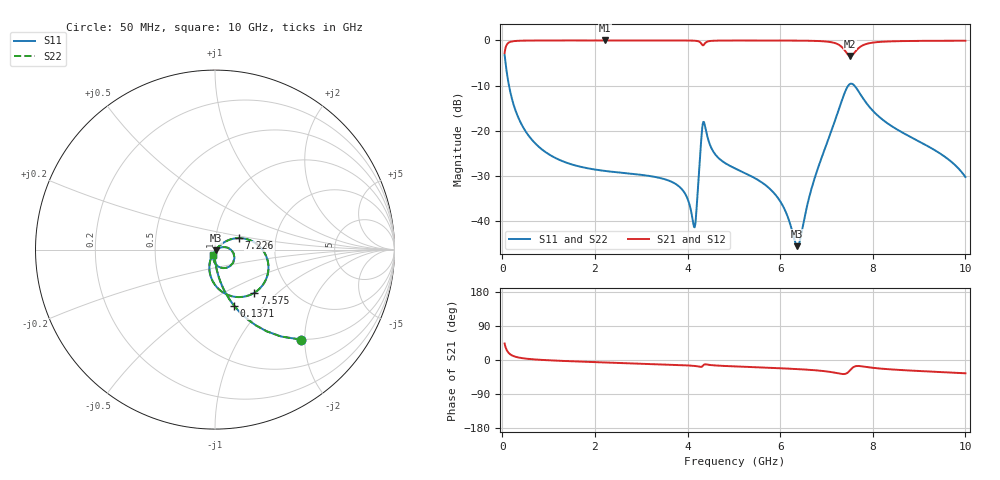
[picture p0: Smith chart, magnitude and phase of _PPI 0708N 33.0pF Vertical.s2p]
! S-Parameter data specifications (vertical orientation):
! Substrate: 40-mil Rogers 3003C, Substrate thickness, H=1.016mm, Dielectric constant, Er=3, Conductor thickness, T_mtl=0.043mm, Loss Tangent, Tand=0.003
! PCB Mounting Pad Footprint: Pad width, PadW=2.54mm , Pad length, PadL=0.51mm , Pad gap, PadG (edge-to-edge)=0.71mm , Reference planes=1.73mm apart
! Created Tue Jan 16 08:53:07 2018
# GHz S MA R 50
! 2 Port Network Data from SP1.SP block
! freq  magS11  angS11  magS21  angS21  magS12  angS12  magS22  angS22
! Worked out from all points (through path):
!   801 points, 50 MHz to 10 GHz, reference 50 ohm
!   highest |S21| = -0.01 dB at 2.214 GHz (marker M1); lowest = -3.5 dB at 7.513 GHz (marker M2)
!   group delay of S21, straight-line fit = 10.8 ps
!   lowest |S11| = -45.6 dB at 6.368 GHz (marker M3), VSWR 1.01, Z = 50.4 - j0.313 ohm
!   |S11| at or under -10 dB: 144 MHz to 7.473 GHz (7.329 GHz wide, 192 % of centre); 7.601 GHz to end of sweep
!   |S22| runs from -45.6 to -3.2 dB; largest |S21 - S12| = 0
!   S11 on the Smith chart (normalised r, x): 50 MHz: 0.99, -1.91; 137.1 MHz: 0.99, -0.70; 7.226 GHz: 1.30, +0.17; 7.575 GHz: 1.34, -0.72; 10 GHz: 0.98, -0.06
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0.05  0.6914 -46.4  0.7223 43.5  0.7223 43.5  0.6914 -46.4
0.1370625  0.3303 -71.2  0.9437 18.8  0.9437 18.8  0.3303 -71.2
0.3360625  0.1433 -83.0  0.9895 6.9  0.9895 6.9  0.1433 -83.0
0.647  0.07833 -87.8  0.9966 2.0  0.9966 2.0  0.07833 -87.8
1.716625  0.03942 -93.7  0.9987 -4.3  0.9987 -4.3  0.03942 -93.7
2.214125  0.03572 -95.7  0.9988 -6.5  0.9988 -6.5  0.03572 -95.7
3.370812  0.03011 -99.7  0.9986 -11.2  0.9986 -11.2  0.03011 -99.7
3.893187  0.02192 -98.9  0.9978 -13.6  0.9978 -13.6  0.02192 -98.9
4.1295  0.009029 -60.9  0.9935 -15.4  0.9935 -15.4  0.009029 -60.9
4.17925  0.01053 -7.2  0.9894 -16.0  0.9894 -16.0  0.01053 -7.2
4.291188  0.07354 7.4  0.933 -18.2  0.933 -18.2  0.07354 7.4
4.353375  0.1247 -48.4  0.8962 -12.4  0.8962 -12.4  0.1247 -48.4
4.602125  0.05417 -99.1  0.9933 -14.4  0.9933 -14.4  0.05417 -99.1
5.025  0.03811 -104.0  0.9971 -16.9  0.9971 -16.9  0.03811 -104.0
5.895625  0.01952 -103.3  0.9969 -21.2  0.9969 -21.2  0.01952 -103.3
6.36825  0.00523 -36.4  0.9946 -24.0  0.9946 -24.0  0.00523 -36.4
6.691625  0.02409 38.9  0.9894 -26.4  0.9894 -26.4  0.02409 38.9
7.226438  0.1491 25.4  0.9166 -34.5  0.9166 -34.5  0.1491 25.4
7.5125  0.3296 -30.8  0.6707 -26.8  0.6707 -26.8  0.3296 -30.8
7.574687  0.3254 -47.7  0.701 -19.5  0.701 -19.5  0.3254 -47.7
8.345812  0.1177 -105.3  0.9744 -24.4  0.9744 -24.4  0.1177 -105.3
10  0.03058 -110.7  0.9915 -35.1  0.9915 -35.1  0.03058 -110.7
